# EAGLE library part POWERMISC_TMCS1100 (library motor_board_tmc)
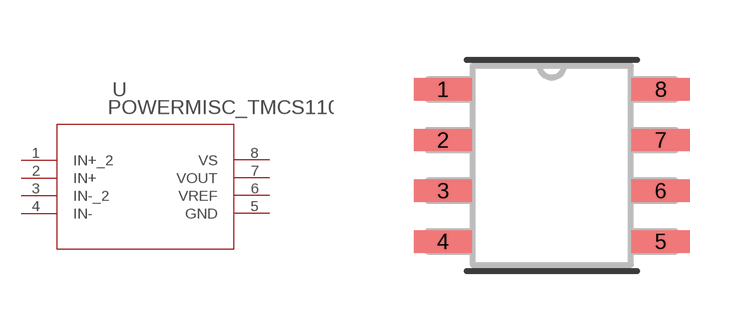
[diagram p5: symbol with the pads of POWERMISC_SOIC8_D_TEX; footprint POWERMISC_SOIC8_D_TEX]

Designator prefix U

## POWERMISC_TMCS1100 (BUILT_BY: EMA_Cory; COPYRIGHT: Copyright (C) 2018 Accelerated Designs. All rights reserved; DATASHEET: https://www.ti.com/lit/ds/symlink/tmcs1100.pdf?ts=1593546414862&ref_url=https%253A%252F%252Fwww.ti.com%252Fproduct%252FTMCS1100; MANUFACTURER_PART_NUMBER: TMCS1100A3QDR; SOURCELIBRARY: TI_2020-06-30; VENDOR: Texas Instruments)  [POWERMISC_SOIC8_D_TEX]
1  IN+_2  in
2  IN+  in
3  IN-_2  in
4  IN-  in
5  GND  pas
6  VREF  pwr
7  VOUT  out
8  VS  pwr

## Footprint POWERMISC_SOIC8_D_TEX (pad centres in mm)
smd 1.46 x 0.559: 1 -2.724,1.905; 2 -2.724,0.635; 3 -2.724,-0.635; 4 -2.724,-1.905; 5 2.724,-1.905; 6 2.724,-0.635; 7 2.724,0.635; 8 2.724,1.905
